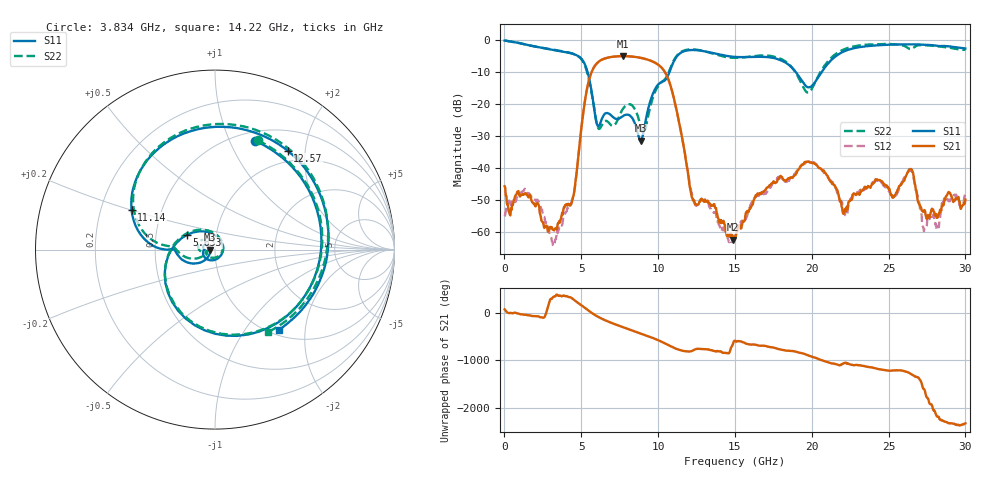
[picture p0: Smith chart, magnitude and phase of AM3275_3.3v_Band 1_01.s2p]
!Keysight Technologies,N5245B,MY58422270,A.16.20.02
!Date: Thursday, March 27, 2025 01:44:15
!Correction: S11(C  2-Port  )
!S21(C  2-Port  )
!S12(C  2-Port  )
!S22(C  2-Port  )
!S2P File: Measurements: S11, S21, S12, S22:
# Hz S  dB  R 50
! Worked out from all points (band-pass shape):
!   801 points, 10 MHz to 30 GHz, reference 50 ohm
!   highest |S21| = -5.13 dB at 7.695 GHz (marker M1); lowest = -62.3 dB at 14.89 GHz (marker M2)
!   |S21| within 3 dB of the highest: 5.89 GHz to 10.09 GHz (4.203 GHz wide, 52.6 % of centre)
!   lowest |S11| = -31.5 dB at 8.857 GHz (marker M3), VSWR 1.05, Z = 47.4 - j0.101 ohm
!   |S11| at or under -10 dB: 5.399 GHz to 10.75 GHz (5.349 GHz wide, 66.3 % of centre); 18.94 GHz to 20.66 GHz (1.715 GHz wide, 8.66 % of centre)
!   |S22| runs from -29.0 to -0.3 dB; largest |S21 - S12| = 0.0052
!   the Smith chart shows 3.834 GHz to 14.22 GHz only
!   S11 on the Smith chart (normalised r, x): 3.834 GHz: 0.60, +1.25; 5.633 GHz: 0.72, +0.12; 11.14 GHz: 0.33, +0.20; 12.57 GHz: 0.81, +1.68; 14.22 GHz: 1.09, -1.45
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1e7  -0.31 -5.1  -45.69 66.1  -55.09 -15.0  -0.26 -5.7
9.097e8  -1.01 -82.6  -47.18 -22.7  -48.12 -15.1  -1.04 -82.9
1.95935e9  -2.13 -161.3  -51.12 -73.6  -49.89 -82.9  -2.13 -162.4
3.833725e9  -3.80 69.7  -52.92 -5.9  -55.23 -2.7  -3.68 68.6
5.033325e9  -6.08 -75.3  -26.40 145.2  -26.40 145.0  -6.30 -78.5
5.633125e9  -15.10 151.9  -10.60 2.8  -10.59 2.7  -15.54 142.7
6.720262e9  -22.91 -153.4  -5.64 175.7  -5.62 175.8  -25.57 -161.9
7.694938e9  -23.89 174.7  -5.13 56.4  -5.14 56.4  -21.70 -174.3
8.85705e9  -31.48 -177.7  -5.67 -75.1  -5.67 -75.1  -26.91 138.8
1.001916e10  -13.94 -167.4  -7.86 140.7  -7.86 140.6  -14.40 -171.9
1.114379e10  -5.76 154.6  -20.71 -32.4  -20.71 -32.4  -5.48 149.0
1.256831e10  -3.30 53.7  -51.47 -37.3  -51.28 -38.9  -3.18 50.3
1.421776e10  -4.86 -51.6  -56.76 -118.4  -58.54 -101.9  -5.25 -57.1
1.489254e10  -5.35 -97.1  -62.34 81.6  -61.74 125.3  -5.69 -104.8
1.5005e10  -5.40 -104.7  -61.36 131.6  -60.42 122.6  -5.70 -112.6
1.747918e10  -5.69 111.1  -44.70 -9.2  -44.49 -8.5  -5.23 106.4
2.002832e10  -14.32 -103.8  -38.48 155.3  -38.30 157.4  -15.12 -118.9
2.175275e10  -4.55 139.2  -48.54 -17.1  -49.24 -11.1  -3.88 131.7
2.501416e10  -1.60 39.6  -46.67 -133.1  -47.26 -133.3  -1.36 36.3
2.643869e10  -1.50 5.2  -40.29 159.7  -40.81 156.7  -2.99 5.1
2.745085e10  -1.62 -21.1  -55.30 51.6  -58.35 -89.6  -1.76 -20.9
3e10  -2.76 -106.6  -49.86 -152.9  -47.76 -147.9  -3.16 -110.4
